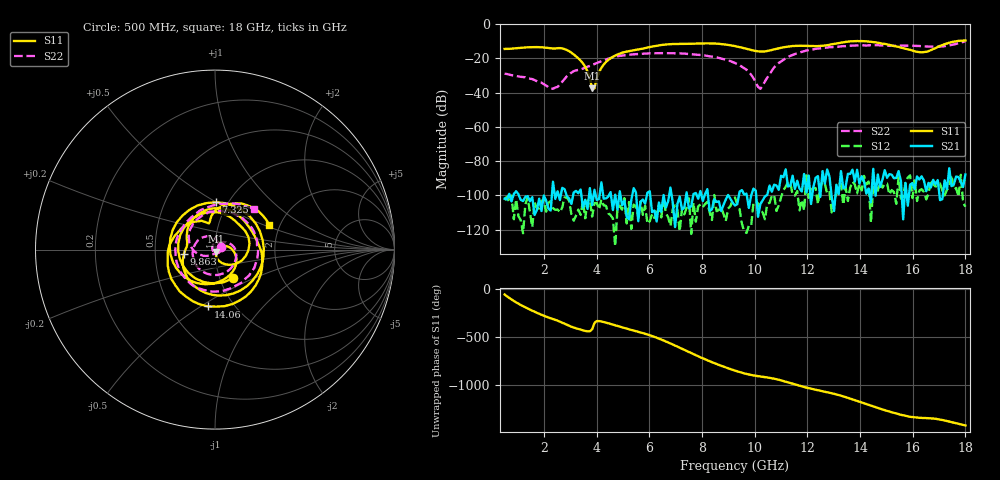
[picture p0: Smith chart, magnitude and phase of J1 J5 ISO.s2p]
!Agilent Technologies,N5230A,MY45001360,A.07.50.67
!Agilent N5230A: A.07.50.67
!Date: Tuesday, April 16, 2024 16:31:16
!Correction: S11(Full 2 Port(1,2))
!S21(Full 2 Port(1,2))
!S12(Full 2 Port(1,2))
!S22(Full 2 Port(1,2))
!S2P File: Measurements: S11, S21, S12, S22:
# Hz S  dB  R 50
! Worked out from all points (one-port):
!   201 points, 500 MHz to 18 GHz, reference 50 ohm
!   lowest |S11| = -37.6 dB at 3.825 GHz (marker M1), VSWR 1.03, Z = 50.7 - j1.14 ohm
!   |S11| at or under -10 dB: start of sweep to 13.74 GHz; 14.16 GHz to 17.66 GHz (3.505 GHz wide, 22 % of centre)
!   S11 on the Smith chart (normalised r, x): 500 MHz: 1.16, -0.38; 7.325 GHz: 0.88, +0.50; 9.863 GHz: 0.70, -0.04; 14.06 GHz: 0.76, -0.54; 18 GHz: 1.76, +0.55
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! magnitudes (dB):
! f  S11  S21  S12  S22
! 500 MHz  -14.5  -101.9  -102.8  -28.9
! 1.55 GHz  -13.4  -101.0  -118.5  -32.1
! 2.337 GHz  -14.3  -92.0  -107.4  -37.7
! 2.862 GHz  -15.1  -100.3  -101.3  -30.5
! 3.475 GHz  -22.9  -107.2  -103.3  -26.0
! 3.65 GHz  -27.7  -107.9  -103.0  -24.9
! 3.825 GHz  -37.6  -105.7  -112.4  -23.8
! 3.913 GHz  -37.5  -96.7  -104.5  -23.3
! 4 GHz  -31.7  -102.7  -104.5  -22.7
! 4.175 GHz  -25.5  -92.4  -102.4  -21.6
! 4.525 GHz  -20.0  -98.1  -111.5  -19.8
! 6.362 GHz  -12.4  -104.2  -105.8  -17.0
! 7.325 GHz  -11.6  -107.1  -111.1  -17.2
! 9.25 GHz  -12.8  -105.9  -101.2  -22.7
! 9.863 GHz  -15.1  -100.1  -117.9  -29.5
! 10.21 GHz  -16.0  -105.1  -108.1  -37.8
! 10.91 GHz  -14.1  -96.8  -105.7  -22.7
! 12.22 GHz  -12.9  -95.2  -95.4  -14.8
! 14.06 GHz  -9.9  -88.8  -97.1  -12.5
! 15.11 GHz  -12.2  -87.6  -99.5  -12.6
! 16.34 GHz  -16.5  -88.9  -96.3  -12.9
! 18 GHz  -9.6  -87.8  -106.6  -10.1
